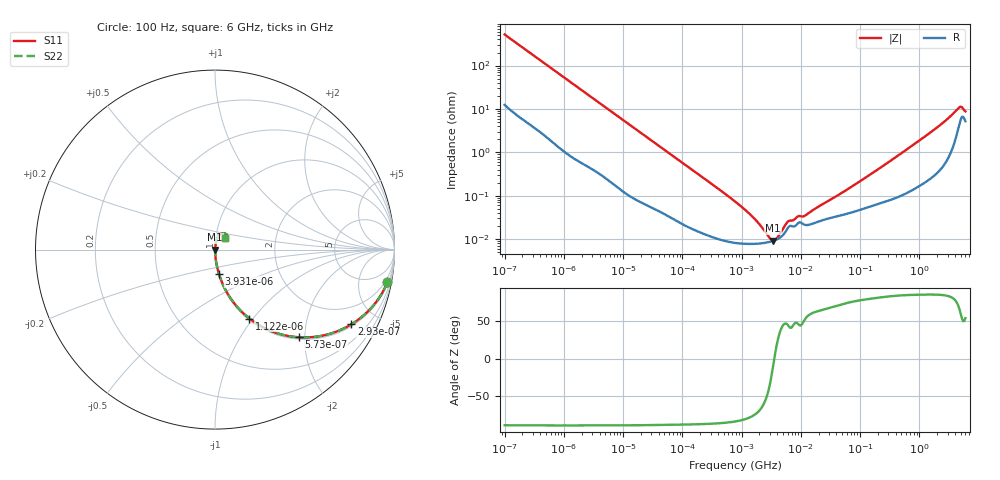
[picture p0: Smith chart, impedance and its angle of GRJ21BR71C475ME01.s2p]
!Murata Part Number: GRJ21BR71C475ME01
!These Parameters are Measured in Series Mode Connection
!Data Generated on Jun 19, 2026
!  o--ll--o
!Port1  Port2
!  o------o
!Operation Temp=25[degC], DC Bias Voltage=0[V]
!Freq. Start=100[Hz] Stop=6[GHz] 401[Steps]
# Hz S RI R 50
!Freq.(Hz) S11(Real) S11(Imag) S21(Real) S21(Imag) S12(Real) S12(Imag) S22(Real) S22(Imag)
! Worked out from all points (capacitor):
!   401 points, 100 Hz to 6 GHz, reference 50 ohm
!   read as one part in series: C = 3.04 uF near 109 Hz
!   lowest |Z| = 9.21 mohm at 3.394 MHz (marker M1)
!   series resonance near 3.572 MHz, so ESL is about 650 pH
!   S11 on the Smith chart (normalised r, x): 100 Hz: 1, -10; 293 Hz: 1.08, -3.61; 573 Hz: 1.04, -1.86; 1.122 kHz: 1.02, -0.96; 3.931 kHz: 1.01, -0.28; 6 GHz: 1.10, +0.14
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100  0.9606 -0.1831  0.0394 0.1831  0.0394 0.1831  0.9606 -0.1831
179  0.8908 -0.3011  0.1092 0.3011  0.1092 0.3011  0.8908 -0.3011
293  0.7605 -0.4159  0.2395 0.4159  0.2395 0.4159  0.7605 -0.4159
573  0.4655 -0.4884  0.5345 0.4884  0.5345 0.4884  0.4655 -0.4884
1122  0.1917 -0.384  0.8083 0.384  0.8083 0.384  0.1917 -0.384
2008  0.0722 -0.2487  0.9278 0.2487  0.9278 0.2487  0.0722 -0.2487
3931  0.022 -0.1356  0.978 0.1356  0.978 0.1356  0.022 -0.1356
10527  0.00393 -0.0524  0.9961 0.0524  0.9961 0.0524  0.00393 -0.0524
40335  0.000634 -0.014  0.9994 0.014  0.9994 0.014  0.000634 -0.014
774597  8.18e-05 -0.00073  0.9999 0.00073  0.9999 0.00073  8.18e-05 -0.00073
1516199  7.72e-05 -0.000322  0.9999 0.000322  0.9999 0.000322  7.72e-05 -0.000322
2837864  8.45e-05 -7.83e-05  0.9999 7.83e-05  0.9999 7.83e-05  8.45e-05 -7.83e-05
3394479  9.04e-05 -1.74e-05  0.9999 1.74e-05  0.9999 1.74e-05  9.04e-05 -1.74e-05
4060267  0.0001 4.41e-05  0.9999 -4.41e-05  0.9999 -4.41e-05  0.0001 4.41e-05
6075234  0.000181 0.000177  0.9998 -0.000177  0.9998 -0.000177  0.000181 0.000177
9090158  0.000235 0.000241  0.9998 -0.000241  0.9998 -0.000241  0.000235 0.000241
1.189169e7  0.000211 0.000278  0.9998 -0.000278  0.9998 -0.000278  0.000211 0.000278
1.555665e7  0.000224 0.000392  0.9998 -0.000392  0.9998 -0.000392  0.000224 0.000392
3.124326e8  0.000817 0.00605  0.9992 -0.00605  0.9992 -0.00605  0.000817 0.00605
1.873145e9  0.00425 0.0346  0.9958 -0.0346  0.9958 -0.0346  0.00425 0.0346
4.586474e9  0.0443 0.0911  0.9557 -0.0911  0.9557 -0.0911  0.0443 0.0911
6e9  0.0538 0.0639  0.9462 -0.0639  0.9462 -0.0639  0.0538 0.0639
